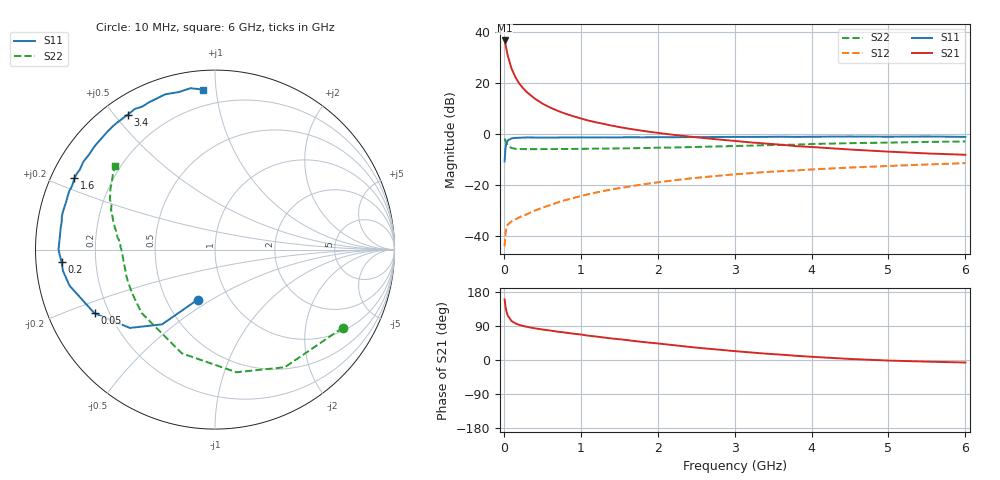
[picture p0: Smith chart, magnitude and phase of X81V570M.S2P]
! SIEMENS Small Signal Semiconductors
! BFP136W
! Si NPN RF Bipolar Junction Transistor in SOT343
! VCE = 1.5 V  IC = 70 mA
! Common Emitter S-Parameters:  September  1994
# GHz  S  MA  R  50
!  f  S11  S21  S12  S22
! GHz  MAG  ANG  MAG  ANG  MAG  ANG  MAG  ANG
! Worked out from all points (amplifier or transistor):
!   40 points, 10 MHz to 6 GHz, reference 50 ohm
!   highest |S21| = 36.9 dB at 10 MHz (marker M1)
!   |S21| within 3 dB of that: start of sweep to 30.81 MHz
!   unconditionally stable (mu >= 1): 513.5 MHz to 2.917 GHz
!   at 200 MHz: K = 0.65, MSG = 26.3 dB, |S12| = -32.6 dB
!   at 1.5 GHz: K = 1.12, MAG = 9.8 dB, |S12| = -21.1 dB
!   at 6 GHz: K = 0.99, MSG = 1.6 dB, |S12| = -11.3 dB
!   S11 on the Smith chart (normalised r, x): 10 MHz: 0.71, -0.44; 50 MHz: 0.15, -0.24; 200 MHz: 0.08, -0.04; 1.6 GHz: 0.07, +0.24; 3.4 GHz: 0.07, +0.54; 6 GHz: 0.10, +0.92
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0.01  0.2952 -109.1  69.79 159.8  0.0064 69.4  0.8347 -31.4
0.02  0.5103 -125.3  59.59 143.2  0.0108 57.5  0.7621 -59.3
0.03  0.6448 -137.4  50.1 131.5  0.0137 46.9  0.6937 -80.1
0.05  0.7594 -152.1  35.57 117.4  0.0169 35.7  0.6067 -107.8
0.1  0.8351 -166.1  19.59 103.0  0.0196 33.2  0.5403 -139.2
0.15  0.8554 -172.0  13.31 96.6  0.0214 35.8  0.5219 -152.2
0.2  0.8579 -175.4  9.977 92.7  0.0235 38.8  0.5168 -159.1
0.25  0.8658 -178.1  8.058 89.8  0.0253 41.6  0.5152 -163.5
0.3  0.8718 180.0  6.73 87.6  0.0271 44.2  0.5128 -166.5
0.4  0.8681 176.6  5.067 83.7  0.0318 49.1  0.5127 -170.5
0.5  0.8673 173.9  4.041 80.5  0.0363 52.3  0.5138 -173.1
0.6  0.8683 172.0  3.372 77.9  0.0409 54.6  0.5147 -174.9
0.7  0.8683 169.6  2.906 74.7  0.0461 56.9  0.5161 -176.2
0.9  0.8732 166.0  2.278 69.6  0.0561 58.8  0.5184 -178.7
1.1  0.8709 161.7  1.866 64.1  0.0669 59.6  0.5226 179.6
1.6  0.8789 153.0  1.312 52.6  0.0931 58.8  0.534 175.7
2.2  0.8793 142.8  0.984 39.3  0.1248 54.6  0.5531 171.0
3.2  0.8938 125.7  0.698 20.1  0.173 45.4  0.6004 162.0
3.4  0.8947 122.9  0.662 16.8  0.1827 43.2  0.6142 160.2
4.5  0.9086 107.8  0.505 2.8  0.2235 33.0  0.6731 150.0
5.5  0.9094 98.6  0.423 -4.3  0.2565 24.9  0.7112 143.0
6  0.8937 94.3  0.398 -6.7  0.2727 20.5  0.7258 139.9
